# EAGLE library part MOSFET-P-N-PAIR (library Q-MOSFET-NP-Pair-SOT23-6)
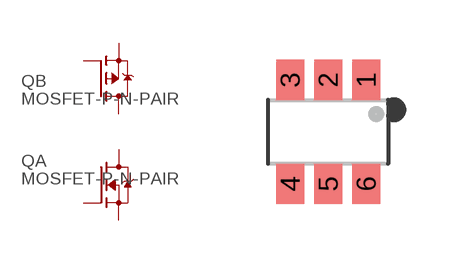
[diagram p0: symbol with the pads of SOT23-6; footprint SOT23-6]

Designator prefix Q; gates A=N-MOSFET B=P-MOSFET

## MOSFET-P-N-PAIR  [SOT23-6]
1  A:G  pas
2  B:S  pas
3  B:G  pas
4  B:D  pas
5  A:S  pas
6  A:D  pas

## Footprint SOT23-6 (pad centres in mm)
SOT23-6 Small Outline Transistor, standard 6-pin package
smd 0.7 x 1: 1 0.95,1.3; 2 0,1.3; 3 -0.95,1.3; 4 -0.95,-1.3; 5 0,-1.3; 6 0.95,-1.3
